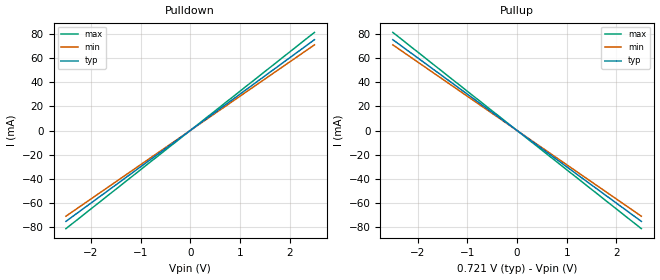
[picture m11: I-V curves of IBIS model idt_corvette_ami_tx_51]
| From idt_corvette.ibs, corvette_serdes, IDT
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|   model   idt_corvette_ami_tx_51
[Model] idt_corvette_ami_tx_51
Model_type Output
C_comp 400f 400f 400f
Cref = 0
[Model Spec]
Vmeas 0. 0. 0.
Vref 0. 0. 0.
[Temperature Range]  25 100 0
[Voltage Range] .721 .706 .686
[Algorithmic Model]
Executable Windows_VisualStudio5_32 idt_corvette_tx.dll   idt_corvette_tx.ami
Executable Windows_ver_64   idt_corvette_tx_64.dll   idt_corvette_tx.ami
Executable Linux_gcc4.1.2_32   idt_corvette_tx.linux.so   idt_corvette_tx.ami
Executable Linux_gcc3.2.3_64   idt_corvette_tx_64.linux.so idt_corvette_tx.ami
[End Algorithmic Model]
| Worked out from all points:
|   slope of the pulldown table from 0 to 0.108 V, typ, clamps not added: 33.1 ohm
|   slope of the pullup table from 0 to 0.108 V, typ, clamps not added: 33.1 ohm
[Pulldown]
-2.5V     -75.43mA   -71.14mA   -81.49mA
0V        0A         0A         0A
2.5V      75.43mA    71.14mA    81.49mA
[Pullup]
-2.5V     75.43mA    71.14mA    81.49mA
0V        0A         0A         0A
2.5V      -75.43mA   -71.14mA   -81.49mA
[Ramp]
dV/dt_r .26/18.56p .249/19.68p .255/17.181p
dV/dt_f .26/18.56p .249/19.68p .255/17.181p
